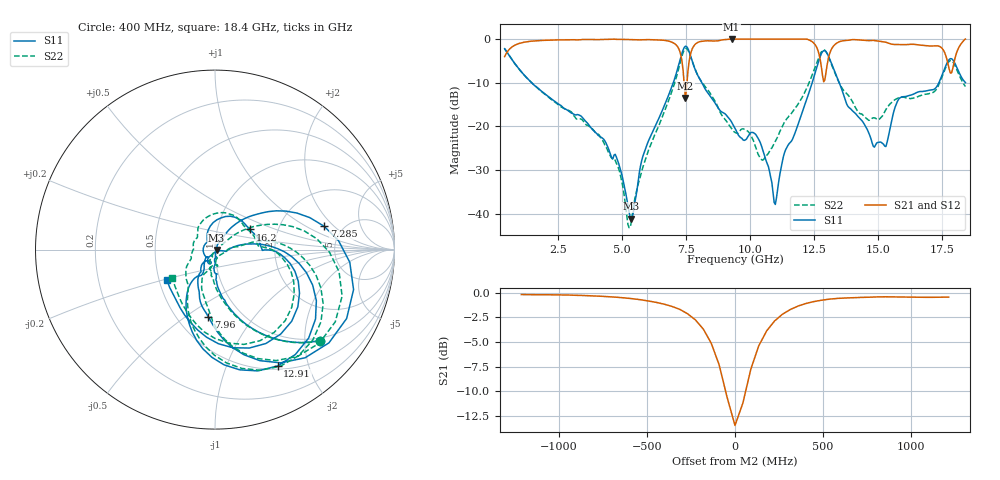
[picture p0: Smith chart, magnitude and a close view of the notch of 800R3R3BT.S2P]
!  American Technical Ceramics  Date:  6/19/09
!  One Norden Lane
!  Huntington Station,  NY.  11746-2102
!  Tel:  (631) 622-4700  Fax:  (631) 622-4748
!  Part Number  800R3R3BT
!  Description: Ultra-low ESR, NPO  Mounting Orientation: Horizontal
!  Application: High RF power Filters, Combiners, Matching networks,
!  Antenna, DC block, Bypass and Couplers
# GHZ S DB R 50
! Freq  |S11|  S11 Ph  |S21|  S21 Ph  |S12|  S12 Ph  |S22|  S22 Ph
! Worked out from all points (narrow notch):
!   401 points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, 400 MHz to 18.4 GHz, reference 50 ohm
!   highest |S21| = -0.01 dB at 9.265 GHz (marker M1); lowest = -13.5 dB at 7.465 GHz (marker M2)
!   notch at M2: 13.2 dB deep, 205 MHz wide at half that depth
!   lowest |S11| = -41.1 dB at 5.35 GHz (marker M3), VSWR 1.02, Z = 50.9 - j0.169 ohm
!   |S11| at or under -10 dB: 1.46 GHz to 6.988 GHz (5.528 GHz wide, 131 % of centre); 8.109 GHz to 12.41 GHz (4.306 GHz wide, 42 % of centre); 13.47 GHz to 17.36 GHz (3.892 GHz wide, 25.2 % of centre)
!   |S22| runs from -43.1 to -2.1 dB; largest |S21 - S12| = 0.0048
!   S11 on the Smith chart (normalised r, x): 400 MHz: 0.93, -2.37; 7.285 GHz: 3.59, +1.52; 7.96 GHz: 0.71, -0.62; 12.91 GHz: 0.54, -1.54; 16.2 GHz: 1.44, +0.34; 18.4 GHz: 0.55, -0.21
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0.4  -2.21 -40.8  -4.02 49.0  -4.04 49.0  -2.21 -41.0
1.3  -9.07 -74.8  -0.59 14.6  -0.61 14.6  -9.10 -75.7
3.415  -17.79 -90.5  -0.13 -7.5  -0.14 -7.4  -18.41 -101.0
4.765  -26.97 -83.8  -0.07 -17.6  -0.08 -17.5  -28.40 -113.3
5.35  -41.13 -10.9  -0.13 -21.8  -0.14 -21.7  -41.86 -15.6
6.43  -18.09 55.2  -0.20 -31.7  -0.20 -31.6  -19.75 37.6
7.285  -4.13 12.1  -3.69 -62.9  -3.69 -62.8  -4.86 6.0
7.465  -1.64 -27.6  -13.49 -30.9  -13.49 -30.8  -2.14 -31.0
7.96  -8.48 -95.6  -0.74 -11.4  -0.73 -11.3  -8.44 -93.2
9.265  -18.98 -131.0  -0.01 -28.5  -0.01 -28.4  -20.46 -101.2
9.4  -20.45 -131.5  -0.01 -29.6  -0.01 -29.5  -21.36 -92.6
10.3  -22.69 -124.6  -0.01 -39.3  -0.01 -39.2  -26.33 -75.7
10.975  -37.84 -59.5  -0.01 -44.5  -0.01 -44.5  -23.41 -2.7
12.415  -10.00 3.0  -0.61 -70.2  -0.60 -70.2  -8.22 3.6
12.91  -2.66 -61.7  -9.34 -40.0  -9.33 -40.0  -2.56 -60.8
13.36  -8.37 -114.6  -0.99 -35.4  -0.98 -35.5  -8.55 -113.5
14.8  -24.51 -136.0  -0.31 -57.8  -0.30 -57.9  -18.02 163.4
15.43  -21.21 120.3  -1.01 -63.2  -1.00 -63.4  -15.02 111.4
16.195  -12.93 29.9  -1.24 -62.8  -1.22 -63.0  -13.53 42.9
17.68  -5.52 -27.2  -4.70 -82.0  -4.69 -82.2  -5.92 -29.2
17.95  -5.10 -79.7  -5.53 -35.8  -5.51 -36.0  -5.58 -81.8
18.4  -9.97 -147.5  -0.01 -44.4  -0.01 -44.6  -10.87 -146.0
